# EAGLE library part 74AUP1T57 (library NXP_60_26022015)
Low-power configurable gate with voltage-level translator The 74AUP1T57 provides low-power, low-voltage configurable logic gate functions. The output state is determined by eight patterns of 3-bit input. The user can choose the logic functions AND, OR, NAND, NOR, XNOR, inverter and buffer. All inputs can be connected to VCC or GND. This device ensures a very low static and dynamic power consumption across the entire VCC range from 2.3 V to 3.6 V. The 74AUP1T57 is designed for logic-level translation applications with input switching levels that accept 1.8 V low-voltage CMOS signals, while operating from either a single 2.5 V or 3.3 V supply voltage. The wide supply voltage range ensures normal operation as battery voltage drops from 3.6 V to 2.3 V. This device is fully specified for partial power-down applications using IOFF. The IOFF circuitry disables the output, preventing the damaging backflow current through the device when it is powered down. Schmitt trigger inputs make the circuit tolerant to slower input rise and fall times across the entire VCC range. AAL Eindhoven MK
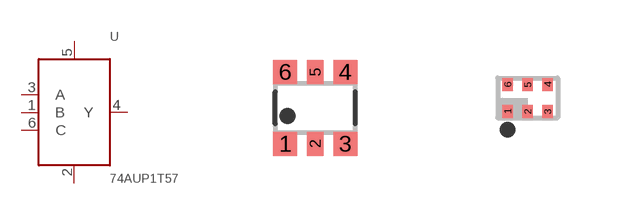
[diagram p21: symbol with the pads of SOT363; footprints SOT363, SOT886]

Designator prefix U

## 74AUP1T57GW (12NC: 9352 804 64125)  [SOT363]
1  B  in
2  GND  pwr
3  A  in
4  Y  out
5  VCC  pwr
6  C  in

## 74AUP1T57GM (12NC: 9352 804 65115)  [SOT886]
Pads as for SOT363

## 74AUP1T57GF (12NC: 9352 813 64132)  [SOT891]
Pads as for SOT363

## 74AUP1T57GS (12NC: 9352 928 78132)  [SOT1202]
Pads as for SOT363

## 74AUP1T57GN (I2C: 9352 917 54132)  [SOT1115]
Pads as for SOT363

## Footprint SOT363 (pad centres in mm)
SOT363 Plastic surface-mounted package; 6 leads JEDEC: -- IEC: -- JEITA: SC-88
smd 0.6 x 0.6: 1 -0.75,-0.9; 3 0.75,-0.9; 4 0.75,0.9; 6 -0.75,0.9
smd 0.4 x 0.6: 2 0,-0.9; 5 0,0.9

## Footprint SOT886 (pad centres in mm)
SOT886 XSON6: plastic extremely thin small outline package; no leads; 6 terminals; body 1 x 1.45 x 0.5 mm JEDEC: MO-252 IEC: ---
smd 0.27 x 0.325: 1 -0.5,-0.338; 2 0,-0.338; 3 0.5,-0.338; 4 0.5,0.338; 5 0,0.338; 6 -0.5,0.338

## Footprint SOT891 (pad centres in mm)
SOT891 XSON6: plastic extremely thin small outline package; no leads; 6 terminals; body 1 x 1 x 0.5 mm JEDEC: -- IEC: ---
smd 0.15 x 0.5: 1 -0.35,-0.35; 2 0,-0.35; 3 0.35,-0.35; 4 0.35,0.35; 5 0,0.35; 6 -0.35,0.35

## Footprint SOT1202 (pad centres in mm)
SOT1202 XSON6: extremely thin small outline package; no leads; 6 terminals; body 1.0 x 1.0 x 0.35 mm JEDEC: --- IEC: ---
smd 0.15 x 0.5: 1 -0.35,-0.35; 2 0,-0.35; 3 0.35,-0.35; 4 0.35,0.35; 5 0,0.35; 6 -0.35,0.35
